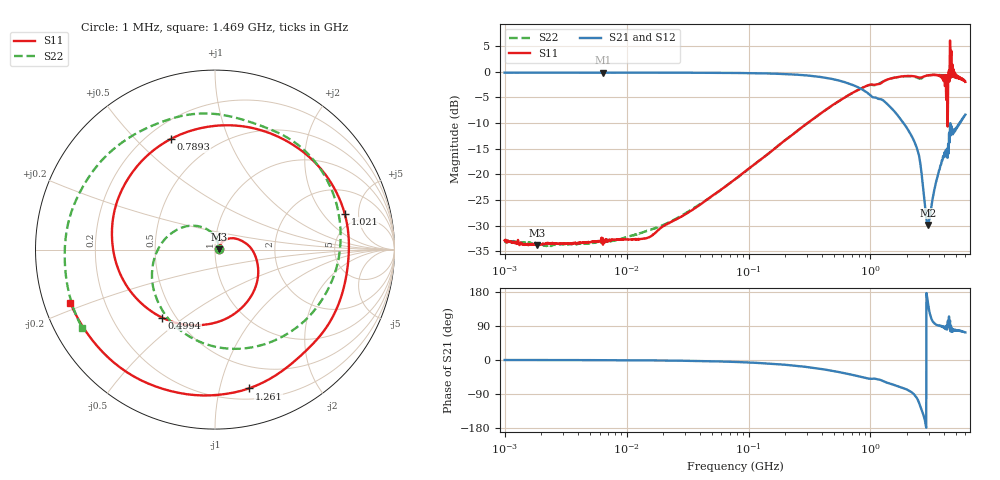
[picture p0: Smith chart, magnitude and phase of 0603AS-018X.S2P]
!s-Parameter Generated by FASTRON Sdn. Bhd.
!FASTRON P/N : 0603AS-018X
!Keysight Technologies: E5071C_MY46733604_B.14.02
!Date: Tue Oct 10 11:12:33 2023
!Version  :Rev01  Tue Oct 10 11:12:33 2023
!Data & Calibration Information:
!Freq  S11:SOLT2(ON)  S21:SOLT2(ON)  S12:SOLT2(ON)  S22:SOLT2(ON)
!PortZ  Port1:50+j0  Port2:50+j0
!When reading reference impedance value at option line is always used.
! Remarks : This data is being provided solely for informational purposes.
# Hz S dB R 50
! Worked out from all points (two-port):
!   1601 points, 1 MHz to 6 GHz, reference 50 ohm
!   highest |S21| = -0.17 dB at 6.378 MHz (marker M1); lowest = -29.8 dB at 2.951 GHz (marker M2)
!   |S21| within 3 dB of the highest: start of sweep to 810.8 MHz
!   lowest |S11| = -33.8 dB at 1.855 MHz (marker M3), VSWR 1.04, Z = 52.1 + j0.194 ohm
!   |S11| at or under -10 dB: start of sweep to 304.5 MHz; 4.289933 GHz to 4.297141 GHz (7.209 MHz wide, 0.168 % of centre)
!   |S22| runs from -34.0 to -0.6 dB; largest |S21 - S12| = 0.0043
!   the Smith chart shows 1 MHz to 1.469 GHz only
!   S11 on the Smith chart (normalised r, x): 1 MHz: 1.05, +0.00; 499.4 MHz: 0.42, -0.42; 789.3 MHz: 0.29, +0.64; 1.021 GHz: 3.76, +3.42; 1.261 GHz: 0.29, -1.23; 1.469 GHz: 0.08, -0.18
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1000000  -32.86 4.8  -0.20 -0.1  -0.19 0.0  -33.03 5.0
1855321  -33.79 5.2  -0.19 -0.1  -0.19 -0.1  -33.53 4.9
4277066  -33.28 11.7  -0.20 -0.3  -0.19 -0.3  -33.45 16.4
6378092  -32.40 15.3  -0.17 -0.4  -0.19 -0.4  -32.97 20.5
1.823719e7  -30.84 35.4  -0.20 -1.3  -0.20 -1.2  -30.21 49.5
7.757876e7  -20.94 40.6  -0.25 -5.1  -0.25 -5.1  -20.98 97.7
3.307917e8  -9.37 -57.7  -0.83 -20.2  -0.83 -20.2  -9.37 -172.2
4.99412e8  -6.37 -127.9  -1.49 -29.2  -1.49 -29.2  -6.38 -117.5
7.892603e8  -3.56 111.9  -3.03 -42.6  -3.04 -42.5  -3.58 -22.5
1.021418e9  -2.50 15.4  -4.83 -49.7  -4.83 -49.6  -2.56 53.4
1.260565e9  -1.98 -76.3  -5.53 -55.5  -5.54 -55.3  -1.94 139.0
1.414819e9  -1.44 -138.0  -6.61 -61.4  -6.61 -61.3  -1.46 -168.1
1.468808e9  -1.32 -159.7  -6.98 -63.1  -6.99 -63.1  -1.32 -149.4
1.981825e9  -0.84 -1.5  -10.91 -77.7  -10.91 -77.6  -0.88 29.8
2.467691e9  -1.11 171.2  -15.80 -107.9  -15.79 -107.8  -1.26 -156.3
2.951149e9  -0.75 -11.3  -29.84 153.5  -29.84 153.5  -0.75 21.9
3.381472e9  -0.61 -175.7  -22.42 95.5  -22.41 95.4  -0.59 177.2
3.867453e9  -1.34 -3.4  -17.31 87.4  -17.31 87.3  -0.75 -6.3
4.353434e9  -0.22 -169.5  -15.63 88.1  -15.62 88.0  -0.73 172.6
4.852826e9  -1.06 -6.6  -11.73 79.9  -11.74 80.0  -0.91 -4.6
5.580302e9  -1.53 81.6  -9.46 76.4  -9.47 76.6  -1.33 -97.4
6e9  -1.99 -75.3  -8.37 72.8  -8.37 73.0  -1.78 56.7
